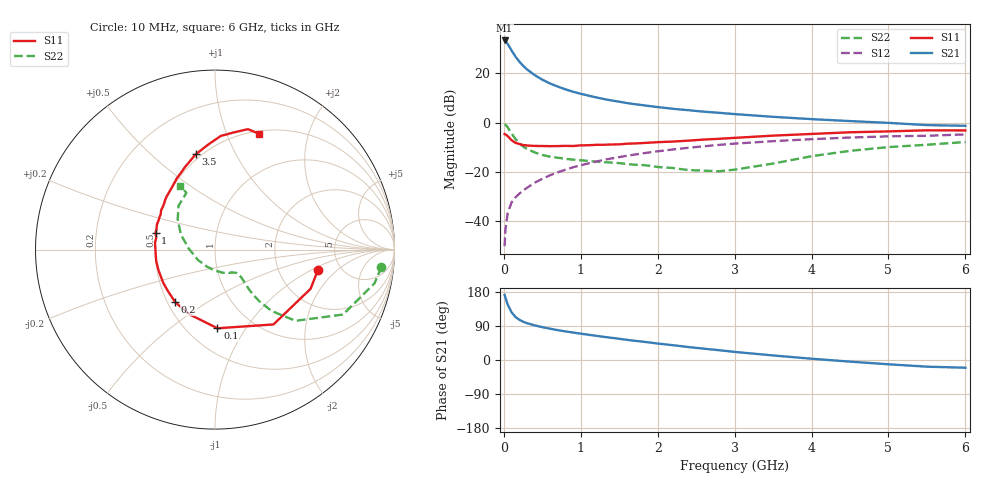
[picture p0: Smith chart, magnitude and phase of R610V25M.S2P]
! SIEMENS Small Signal Semiconductors
! BFR193
! Si NPN RF Bipolar Junction Transistor in SOT23
! VCE = 10 V  IC = 25 mA
! Common Emitter S-Parameters:  May  1996
# GHz  S  MA  R  50
!  f  S11  S21  S12  S22
! GHz  MAG  ANG  MAG  ANG  MAG  ANG  MAG  ANG
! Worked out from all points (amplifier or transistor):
!   36 points, 10 MHz to 6 GHz, reference 50 ohm
!   highest |S21| = 33.3 dB at 10 MHz (marker M1)
!   |S21| within 3 dB of that: start of sweep to 80.71 MHz
!   unconditionally stable (mu >= 1): 556.1 MHz to 2.133 GHz
!   at 250 MHz: K = 0.85, MSG = 25.3 dB, |S12| = -27.6 dB
!   at 1.4 GHz: K = 1.03, MAG = 10.8 dB, |S12| = -14.6 dB
!   at 6 GHz: K = 0.94, MSG = 1.7 dB, |S12| = -4.8 dB
!   S11 on the Smith chart (normalised r, x): 10 MHz: 3.37, -1.17; 100 MHz: 0.69, -0.75; 200 MHz: 0.55, -0.37; 1 GHz: 0.50, +0.11; 3.5 GHz: 0.47, +0.70; 6 GHz: 0.53, +1.31
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0.01  0.5846 -11.3  46.25 171.9  0.0031 75.3  0.9325 -5.9
0.02  0.5757 -22.3  44.87 164.7  0.0066 73.4  0.9088 -11.9
0.05  0.5292 -52.0  39.46 146.4  0.0145 70.0  0.7996 -26.9
0.1  0.4385 -88.2  29.12 125.9  0.0238 62.8  0.5988 -41.5
0.15  0.3877 -112.0  21.88 113.8  0.0303 62.0  0.4654 -47.3
0.2  0.3669 -127.3  17.34 106.3  0.0359 63.5  0.3827 -49.3
0.25  0.3492 -139.0  14.18 101.1  0.0415 64.8  0.3267 -49.8
0.3  0.3425 -147.6  12 97.2  0.0472 66.3  0.2919 -49.5
0.4  0.3351 -160.0  9.197 91.5  0.06 68.1  0.2477 -48.1
0.5  0.3338 -169.0  7.394 86.6  0.0718 69.0  0.2194 -46.8
0.6  0.3315 -176.1  6.213 82.6  0.0849 69.0  0.2031 -46.4
0.7  0.3329 178.0  5.372 78.8  0.0977 69.3  0.1929 -46.4
0.8  0.3363 173.3  4.712 75.5  0.1102 68.2  0.1835 -47.0
1  0.3442 164.0  3.826 69.5  0.1358 67.0  0.1713 -48.6
1.1  0.346 160.3  3.508 66.6  0.1487 66.1  0.1663 -50.8
1.6  0.3719 143.8  2.482 53.2  0.2115 60.3  0.1437 -63.3
2.2  0.4108 128.1  1.898 39.0  0.2844 52.3  0.1192 -87.9
2.8  0.4677 114.0  1.573 25.8  0.3521 43.6  0.1026 -132.1
3.5  0.542 101.4  1.305 12.0  0.4187 32.9  0.147 177.4
4.5  0.634 87.1  1.07 -4.3  0.4964 19.1  0.2664 141.3
5.5  0.6957 74.7  0.886 -17.6  0.5385 5.3  0.3545 116.7
6  0.6909 69.3  0.858 -20.4  0.5739 1.3  0.4018 118.6
